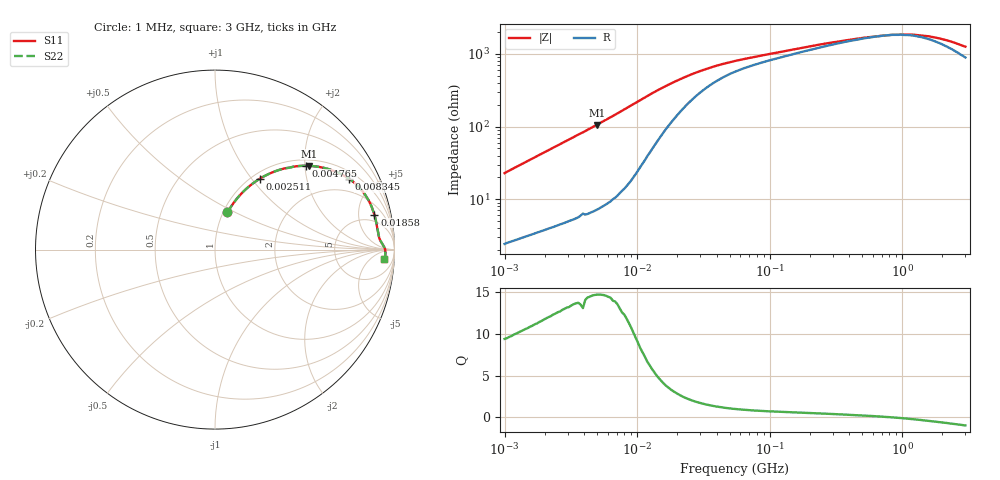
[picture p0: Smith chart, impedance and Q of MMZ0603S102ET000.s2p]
! S-Parameter Data Generated by TDK Corporation
! Copyright(C) 2025 TDK Corporation.
! All Rights Reserved.
! TDK P/N: MMZ0603S102ET000 (Chip Bead)
! Property: |Z|=1000ohm at 100MHz
! Size(LxWxT): 0.6x0.3x0.3mm
! Model Type: s2p (Touchstone File Format Version 1.0)
! Frequency: DC=Yes Start=1MHz Stop=3000MHz 202points Log-sweep
! Model Generated on Feb. 6, 2025
! Terms and conditions regarding TDK Simulation Models:
! 1)This simulation model is being provided solely for informational
!  purposes. Please refer to the specifications of the products in
!  terms of detailed characteristics of such products.
! 2)In no event shall TDK Corporation of any of its subsidiaries be
!  liable for any loss or damage arising, directly or indirectly,
!  from any information contained in this simulation model, including,
!  but not limited to loss or damages arising from any inaccuracies,
!  omissions or errors in connection with such information.
! 3)Any and all copyrights on this simulation model are owned by
!  TDK Corporation.  Duplication or redistribution of this simulation
!  model without prior written permission from TDK Corporation
!  is prohibited.
! 4)This simulation model is subject to any modification or change
!  without any prior notice.
! 5)Neither TDK Corporation nor any of its subsidiaries shall make any
!  warranty, express or implied, including but not limited to the
!  correctness, implied warranties of merchantability and fitness for
!  a particular purpose with respect to this simulation models.
! 6)The use of this simulation model shall be deemed to have consented
!  to the terms and conditions hereof.
! Port Assignments:
!  1 ---@@@--- 2
! Applicable Conditions:
!  Temperature = 25 degC
!  DC Bias Current = 0 A
!  Small Signal Operation
# Hz S MA R 50
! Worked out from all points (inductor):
!   201 points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, 1 MHz to 3 GHz, reference 50 ohm
!   read as one part in series: L = 3.6 uH near 1.041 MHz
!   highest Q = 14.7 at 4.959 MHz (marker M1), where L = 3.38 uH
!   self-resonance near 810.8 MHz
!   S11 on the Smith chart (normalised r, x): 1 MHz: 1.05, +0.46; 2.511 MHz: 1.09, +1.10; 4.765 MHz: 1.14, +2.03; 8.345 MHz: 1.30, +3.60; 18.58 MHz: 3.44, +7.71; 3 GHz: 19, -18
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1000000  0.2183 71.4  0.9531 -12.5  0.9531 -12.5  0.2183 71.4
1616692  0.3317 65.5  0.9138 -19.3  0.9138 -19.3  0.3317 65.5
2055611  0.4018 61.6  0.8826 -23.6  0.8826 -23.6  0.4018 61.6
2511129  0.4668 57.7  0.8482 -27.7  0.8482 -27.7  0.4668 57.7
3323290  0.5643 51.5  0.7852 -34.2  0.7852 -34.2  0.5643 51.5
3900413  0.6175 47.6  0.741 -38.0  0.741 -38.0  0.6175 47.6
4764734  0.6895 42.6  0.679 -43.5  0.679 -43.5  0.6895 42.6
4959344  0.7029 41.6  0.6653 -44.5  0.6653 -44.5  0.7029 41.6
6305767  0.7772 35.2  0.5776 -50.8  0.5776 -50.8  0.7772 35.2
8345207  0.8449 27.8  0.4683 -57.3  0.4683 -57.3  0.8449 27.8
1.104425e7  0.8861 21.1  0.3635 -61.5  0.3635 -61.5  0.8861 21.1
1.461624e7  0.9038 15.8  0.2787 -62.1  0.2787 -62.1  0.9038 15.8
1.858443e7  0.909 12.4  0.2248 -60.1  0.2248 -60.1  0.909 12.4
3.127247e7  0.9119 7.4  0.152 -50.9  0.152 -50.9  0.9119 7.4
5.477226e7  0.9156 4.6  0.1141 -40.1  0.1141 -40.1  0.9156 4.6
2.136344e8  0.935 1.8  0.07173 -24.1  0.07173 -24.1  0.935 1.8
4.75755e8  0.944 0.7  0.05738 -12.1  0.05738 -12.1  0.944 0.7
8.005644e8  0.9481 0.0  0.05194 -0.4  0.05194 -0.4  0.9481 0.0
1.147801e9  0.9499 -0.6  0.05111 10.9  0.05111 10.9  0.9499 -0.6
1.581072e9  0.9502 -1.2  0.05411 22.4  0.05411 22.4  0.9502 -1.2
2.177892e9  0.949 -2.0  0.06141 32.9  0.06141 32.9  0.949 -2.0
3e9  0.9454 -3.0  0.07489 41.7  0.07489 41.7  0.9454 -3.0
